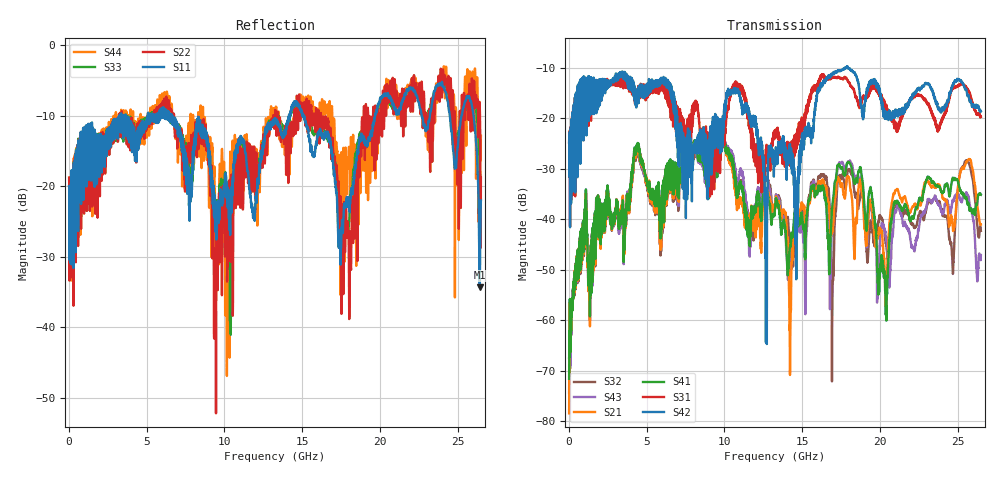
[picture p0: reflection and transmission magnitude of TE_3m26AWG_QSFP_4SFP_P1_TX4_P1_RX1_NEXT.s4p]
!Agilent Technologies,N5222A,MY51421691,A.10.00.00
!Agilent N5222A: A.10.00.00
!Date: Friday, January 30, 2015 12:34:03
!Correction: S11(Full 4 Port(1,2,3,4))
!S12(Full 4 Port(1,2,3,4))
!S13(Full 4 Port(1,2,3,4))
!S14(Full 4 Port(1,2,3,4))
!S21(Full 4 Port(1,2,3,4))
!S22(Full 4 Port(1,2,3,4))
!S23(Full 4 Port(1,2,3,4))
!S24(Full 4 Port(1,2,3,4))
!S31(Full 4 Port(1,2,3,4))
!S32(Full 4 Port(1,2,3,4))
!S33(Full 4 Port(1,2,3,4))
!S34(Full 4 Port(1,2,3,4))
!S41(Full 4 Port(1,2,3,4))
!S42(Full 4 Port(1,2,3,4))
!S43(Full 4 Port(1,2,3,4))
!S44(Full 4 Port(1,2,3,4))
!S4P File: Measurements: <S11,S12,S13,S14>,
!<S21,S22,S23,S24>,
!<S31,S32,S33,S34>,
!<S41,S42,S43,S44>:
# Hz S  dB  R 50.0
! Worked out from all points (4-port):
!   2650 points, 10 MHz to 26.5 GHz, reference 50 ohm
!   strongest paths, dB at 10 MHz, 6.63 GHz, 13.26 GHz, 19.88 GHz, 26.5 GHz:
!     S42: -24.8, -16.1, -29.4, -13.3, -18.6
!     S31: -24.7, -19.1, -23.3, -14.9, -19.7
!     S41: -71.6, -28.7, -38.0, -52.5, -35.1
!     S21: -78.5, -29.1, -37.9, -43.3, -41.0
!     S43: -67.6, -29.2, -37.2, -51.8, -47.1
!     S32: -74.4, -29.6, -37.6, -41.3, -42.3
!   lowest |S11| = -34.3 dB at 26.43 GHz (marker M1), VSWR 1.04, Z = 51.4 - j1.38 ohm
!   |S11| at or under -10 dB: start of sweep to 3.24 GHz; 6.606 GHz to 14.16 GHz (7.55 GHz wide, 72.7 % of centre); 15.11 GHz to 19.69 GHz (4.576 GHz wide, 26.3 % of centre)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
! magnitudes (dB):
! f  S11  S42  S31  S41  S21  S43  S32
! 10 MHz  -20.0  -24.8  -24.7  -71.6  -78.5  -67.6  -74.4
! 4.38 GHz  -13.0  -14.6  -14.8  -25.2  -25.6  -25.3  -25.7
! 10.84 GHz  -14.6  -14.1  -14.1  -35.7  -37.8  -33.6  -35.3
! 12.68 GHz  -12.0  -45.4  -27.0  -34.9  -34.7  -32.0  -32.2
! 17.08 GHz  -18.6  -11.0  -11.8  -33.1  -36.6  -34.9  -41.9
! 26.43 GHz  -34.3  -18.4  -19.4  -34.9  -40.7  -47.2  -42.2
! 26.5 GHz  -22.0  -18.6  -19.7  -35.1  -41.0  -47.1  -42.3
